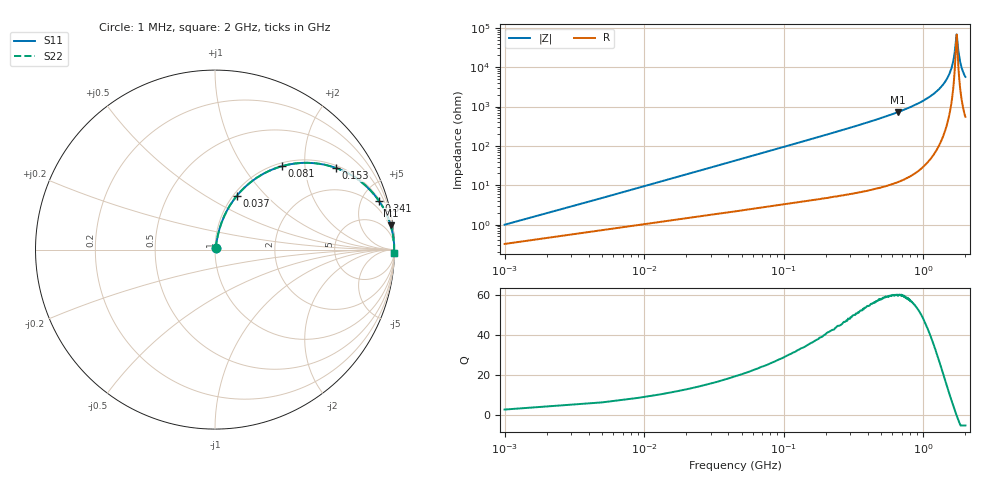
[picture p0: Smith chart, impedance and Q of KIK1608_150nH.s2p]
!version-2
!date-01.2022
!Series
# MHz S RI R 50
!Freq ReS11 ImS11 ReS21 ImS21 ReS12 ImS12 ReS22 ImS22
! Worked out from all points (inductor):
!   501 points, 1 MHz to 2 GHz, reference 50 ohm
!   read as one part in series: L = 150 nH near 9 MHz
!   highest Q = 60 at 657 MHz (marker M1), where L = 175 nH
!   self-resonance near 1.73 GHz
!   S11 on the Smith chart (normalised r, x): 1 MHz: 1.01, +0.02; 37 MHz: 1.04, +0.70; 81 MHz: 1.06, +1.53; 153 MHz: 1.08, +2.91; 341 MHz: 1.13, +6.69; 2 GHz: open
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1  0.00333 0.00936  0.9967 -0.00936  0.9967 -0.00936  0.00333 0.00936
13  0.0259 0.118  0.9741 -0.118  0.9741 -0.118  0.0259 0.118
17  0.0373 0.1522  0.9627 -0.1522  0.9627 -0.1522  0.0373 0.1522
37  0.1221 0.3003  0.8779 -0.3003  0.8779 -0.3003  0.1221 0.3003
81  0.3742 0.4651  0.6258 -0.4651  0.6258 -0.4651  0.3742 0.4651
153  0.6743 0.4548  0.3257 -0.4548  0.3257 -0.4548  0.6743 0.4548
229  0.8227 0.3704  0.1773 -0.3704  0.1773 -0.3704  0.8227 0.3704
337  0.9115 0.2744  0.0885 -0.2744  0.0885 -0.2744  0.9115 0.2744
341  0.9135 0.2716  0.0865 -0.2716  0.0865 -0.2716  0.9135 0.2716
657  0.9791 0.1351  0.0209 -0.1351  0.0209 -0.1351  0.9791 0.1351
669  0.98 0.132  0.02 -0.132  0.02 -0.132  0.98 0.132
1003  0.9937 0.0696  0.00634 -0.0696  0.00634 -0.0696  0.9937 0.0696
1337  0.9977 0.0317  0.00233 -0.0317  0.00233 -0.0317  0.9977 0.0317
1550  0.9985 0.0135  0.00155 -0.0135  0.00155 -0.0135  0.9985 0.0135
1610  0.9985 0.00888  0.00147 -0.00888  0.00147 -0.00888  0.9985 0.00888
1670  0.9986 0.00442  0.00145 -0.00442  0.00145 -0.00442  0.9986 0.00442
1720  0.9985 0.000689  0.00146 -0.000689  0.00146 -0.000689  0.9985 0.000689
1733  0.9985 -0.000157  0.00147 0.000157  0.00147 0.000157  0.9985 -0.000157
1780  0.9985 -0.00348  0.00151 0.00348  0.00151 0.00348  0.9985 -0.00348
1840  0.9984 -0.00751  0.0016 0.00751  0.0016 0.00751  0.9984 -0.00751
1920  0.9982 -0.0127  0.00178 0.0127  0.00178 0.0127  0.9982 -0.0127
2000  0.998 -0.0174  0.00199 0.0174  0.00199 0.0174  0.998 -0.0174
